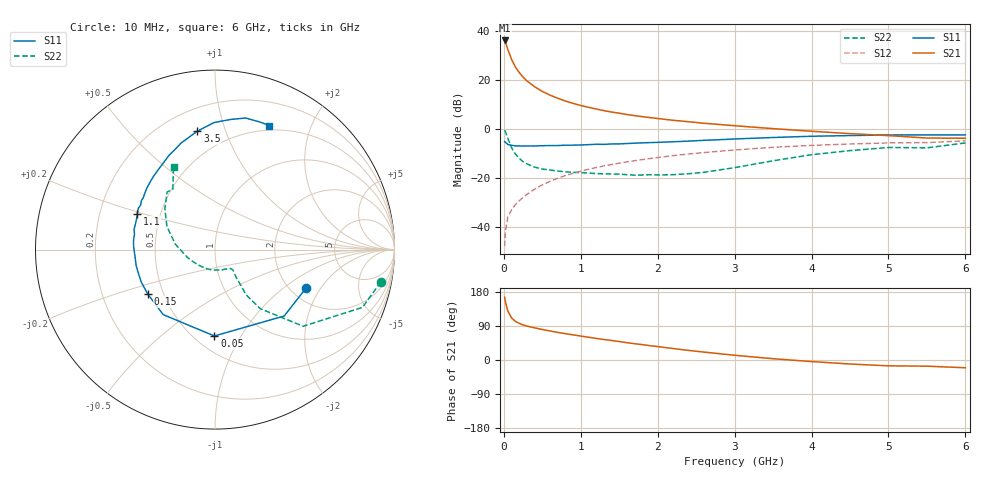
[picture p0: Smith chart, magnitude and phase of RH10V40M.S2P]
! SIEMENS Small Signal Semiconductors
! BFR106
! Si NPN RF Bipolar Junction Transistor in SOT23
! VCE = 10 V  IC = 40 mA
! Common Emitter S-Parameters:  August  1996
# GHz  S  MA  R  50
!  f  S11  S21  S12  S22
! GHz  MAG  ANG  MAG  ANG  MAG  ANG  MAG  ANG
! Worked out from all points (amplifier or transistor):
!   36 points, 10 MHz to 6 GHz, reference 50 ohm
!   highest |S21| = 36.2 dB at 10 MHz (marker M1)
!   |S21| within 3 dB of that: start of sweep to 44.42 MHz
!   unconditionally stable (mu >= 1): 283.7 MHz to 2.269 GHz
!   at 250 MHz: K = 0.97, MSG = 24.6 dB, |S12| = -28.0 dB
!   at 1.4 GHz: K = 1.06, MAG = 9.2 dB, |S12| = -14.6 dB
!   at 6 GHz: K = 0.98, MSG = 0.5 dB, |S12| = -4.9 dB
!   S11 on the Smith chart (normalised r, x): 10 MHz: 2.41, -1.48; 50 MHz: 0.62, -0.78; 150 MHz: 0.41, -0.25; 1.1 GHz: 0.37, +0.19; 3.5 GHz: 0.34, +0.81; 6 GHz: 0.45, +1.44
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0.01  0.5504 -23.0  64.41 165.7  0.004 82.8  0.9418 -11.0
0.02  0.5343 -43.8  59.8 154.3  0.0079 73.3  0.8822 -21.4
0.05  0.4812 -90.4  42.86 129.8  0.0155 62.8  0.651 -41.0
0.1  0.4632 -128.5  26.48 111.3  0.0221 58.5  0.415 -52.5
0.15  0.4489 -146.7  18.48 101.9  0.0283 60.4  0.3064 -55.5
0.2  0.4489 -156.4  14.23 96.6  0.0339 63.7  0.2513 -54.3
0.25  0.4468 -163.8  11.44 92.5  0.0399 65.3  0.2132 -53.3
0.3  0.4482 -168.8  9.601 89.6  0.0458 67.3  0.1929 -52.6
0.4  0.4475 -176.0  7.282 84.8  0.0587 69.2  0.1654 -50.3
0.5  0.4536 178.2  5.846 80.5  0.0716 70.0  0.1512 -48.6
0.6  0.4568 173.2  4.91 76.6  0.0845 69.9  0.1443 -49.2
0.7  0.4567 169.3  4.238 72.8  0.0978 69.8  0.1375 -50.6
0.9  0.4654 162.2  3.326 66.3  0.124 68.1  0.1294 -52.9
1.1  0.4768 155.4  2.768 60.1  0.1495 66.3  0.1252 -60.1
1.3  0.4828 149.2  2.366 54.1  0.175 63.9  0.1205 -66.3
1.6  0.5029 140.8  1.968 45.7  0.2116 60.4  0.1159 -80.0
2.2  0.5459 125.5  1.501 30.3  0.2838 52.4  0.116 -114.1
2.8  0.6011 111.7  1.233 16.7  0.3498 43.9  0.1447 -154.9
3.5  0.6676 98.4  1.013 3.4  0.4205 33.8  0.2231 172.2
4.5  0.7306 83.1  0.8 -10.6  0.4913 19.1  0.36 140.9
5.5  0.7535 70.6  0.651 -16.3  0.5249 8.7  0.4101 125.0
6  0.755 66.3  0.644 -20.5  0.5691 1.6  0.5172 116.5
